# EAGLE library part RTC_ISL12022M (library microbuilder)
Temp. Compensated +/-5ppm RTC
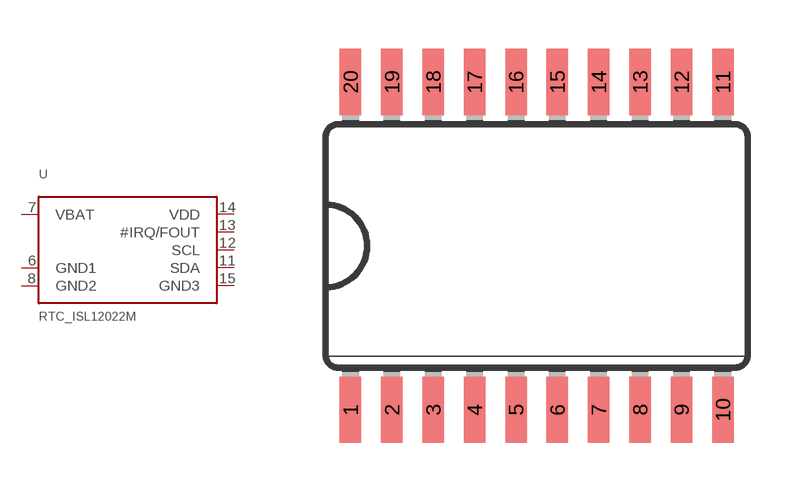
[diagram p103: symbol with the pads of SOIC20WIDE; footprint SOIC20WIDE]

Designator prefix U

## RTC_ISL12022M  [SOIC20WIDE]
6  GND1  pwr
7  VBAT  pwr
8  GND2  pwr
11  SDA
12  SCL
13  #IRQ/FOUT
14  VDD  pwr
15  GND3  pwr

## Footprint SOIC20WIDE (pad centres in mm)
smd 0.66 x 2.032: 1 -5.715,-5.029; 2 -4.445,-5.029; 3 -3.175,-5.029; 4 -1.905,-5.029; 5 -0.635,-5.029; 6 0.635,-5.029; 7 1.905,-5.029; 8 3.175,-5.029; 9 4.445,-5.029; 10 5.715,-5.029; 11 5.715,5.029; 12 4.445,5.029; 13 3.175,5.029; 14 1.905,5.029; 15 0.635,5.029; 16 -0.635,5.029; 17 -1.905,5.029; 18 -3.175,5.029; 19 -4.445,5.029; 20 -5.715,5.029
